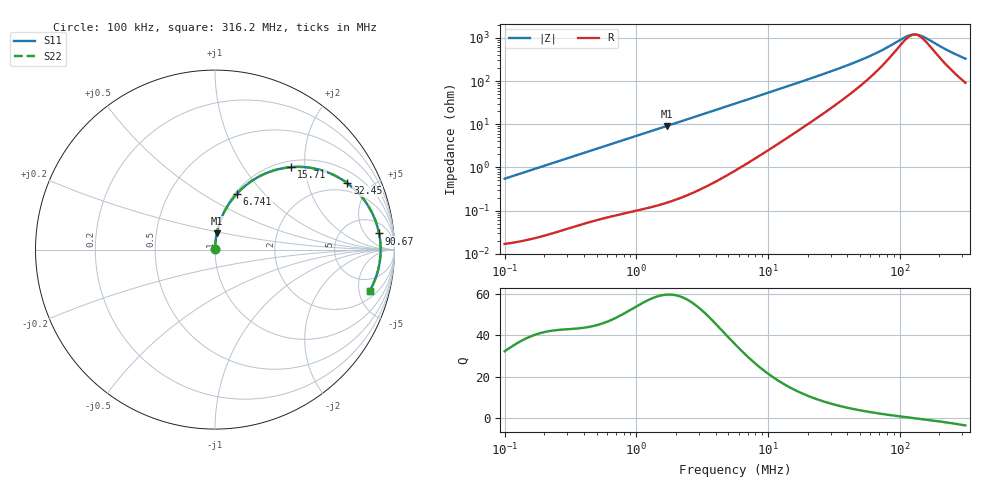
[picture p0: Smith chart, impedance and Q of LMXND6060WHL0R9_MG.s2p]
! LMXND6060WHL0R9_MG  S-PARAMETER MODEL  ( General Type )
! Model Generated by TAIYO YUDEN Corporation (https://www.yuden.co.jp/en/)
! Version 1.0
! TAIYO YUDEN Control No. 191025NI43SB-FBB
! Copyright(c) 2019 TAIYO YUDEN CO.,LTD. All Rights Reserved.
! Product Description (link to TY-COMPAS)
! https://ds.yuden.co.jp/TYCOMPAS/or/detail?pn=LMXND6060WHL0R9NMG&u=M
! Products Name : Inductors
! Characteristics :
!  Inductance : 0.90 uH , SRF(min) : 90 MHz , DC Resistance(max) : 0.0169 Ohm
!  Rated Current : Saturation :6700 mA , Temp Rise : 4600 mA (40 degC)
!  Case Size : 6.0 x 6.0 / 0.236 x 0.236 [mm/inch] , Thickness : 2.8 / 0.11 [mm/inch]
!  (Conditions: Temperature = 25 degC , DC Bias Current/Voltage = 0A / 0V)
! External Node Assignments :
!  1  o---GGG---o  2
! GND o---------o GND
! Frequency Range : 0.1MHz  -  316.199832MHz  [ 402 STEP ]
# MHz S RI R 50
! Freq[MHz].  S11 Real  S11 Imag  S21 Real  S21 Imag  S12 Real  S12 Imag  S22 Real  S22 Imag
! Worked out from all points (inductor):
!   401 points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, 100 kHz to 316.2 MHz, reference 50 ohm
!   read as one part in series: L = 872 nH near 104.1 kHz
!   highest Q = 59.7 at 1.713 MHz (marker M1), where L = 850 nH
!   self-resonance near 130.3 MHz
!   S11 on the Smith chart (normalised r, x): 100 kHz: 1.00, +0.01; 6.741 MHz: 1.02, +0.72; 15.71 MHz: 1.12, +1.69; 32.45 MHz: 1.56, +3.60; 90.67 MHz: 10, +12; 316.2 MHz: 2.83, -6.36
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0.1  0.000199 0.00548  0.9998 -0.00548  0.9998 -0.00548  0.000199 0.00548
0.385695  0.000916 0.0209  0.9991 -0.0209  0.9991 -0.0209  0.000916 0.0209
1.487603  0.00759 0.0788  0.9924 -0.0788  0.9924 -0.0788  0.00759 0.0788
1.712918  0.00978 0.0904  0.9902 -0.0904  0.9902 -0.0904  0.00978 0.0904
3.134972  0.0301 0.1616  0.9699 -0.1616  0.9699 -0.1616  0.0301 0.1616
5.623165  0.089 0.271  0.911 -0.271  0.911 -0.271  0.089 0.271
6.741087  0.1225 0.3121  0.8775 -0.3121  0.8775 -0.3121  0.1225 0.3121
10.08621  0.2361 0.402  0.7639 -0.402  0.7639 -0.402  0.2361 0.402
15.7118  0.4233 0.4595  0.5767 -0.4595  0.5767 -0.4595  0.4233 0.4595
21.68824  0.5757 0.4468  0.4243 -0.4468  0.4243 -0.4468  0.5757 0.4468
32.45058  0.7379 0.3694  0.2621 -0.3694  0.2621 -0.3694  0.7379 0.3694
42.16686  0.813 0.299  0.187 -0.299  0.187 -0.299  0.813 0.299
54.79236  0.8645 0.225  0.1355 -0.225  0.1355 -0.225  0.8645 0.225
68.38627  0.893 0.1639  0.107 -0.1639  0.107 -0.1639  0.893 0.1639
83.65039  0.9096 0.1107  0.0904 -0.1107  0.0904 -0.1107  0.9096 0.1107
90.67083  0.9142 0.0901  0.0858 -0.0901  0.0858 -0.0901  0.9142 0.0901
117.8193  0.9224 0.0247  0.0776 -0.0247  0.0776 -0.0247  0.9224 0.0247
127.7074  0.923 0.00489  0.077 -0.00489  0.077 -0.00489  0.923 0.00489
138.4253  0.9228 -0.0149  0.0772 0.0149  0.0772 0.0149  0.9228 -0.0149
156.2122  0.9209 -0.0447  0.0791 0.0447  0.0791 0.0447  0.9209 -0.0447
243.3397  0.895 -0.1586  0.105 0.1586  0.105 0.1586  0.895 -0.1586
316.1998  0.8612 -0.2308  0.1388 0.2308  0.1388 0.2308  0.8612 -0.2308
